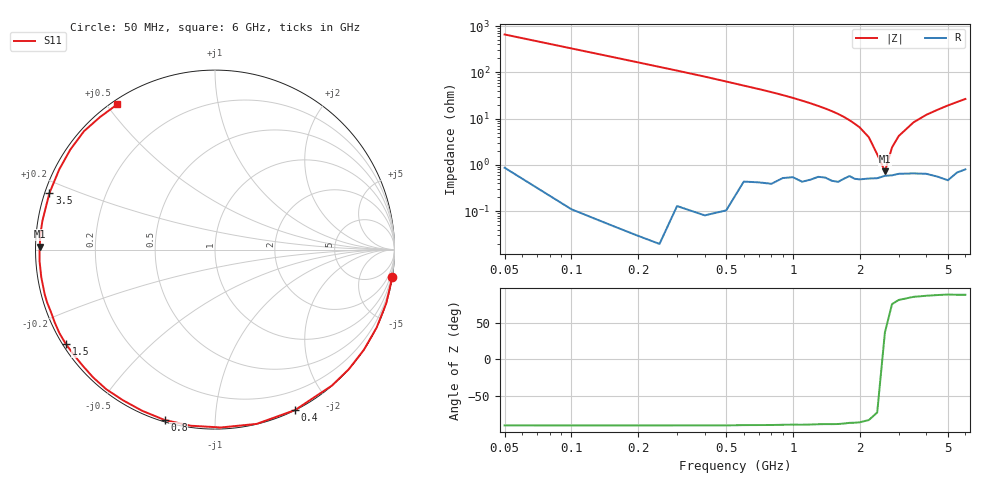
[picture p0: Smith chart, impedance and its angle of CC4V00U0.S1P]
! Infineon Technologies  Discrete & RF Semiconductors
! BBY57-02W
! Si Tuning Diode in SCD-80
! VR = 4 V
! S-Parameters:  June  2000
# GHz  S  MA  R  50
!  f  S11
! GHz  MAG  ANG
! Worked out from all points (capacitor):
!   34 points, 50 MHz to 6 GHz, reference 50 ohm
!   read as one part to ground: C = 4.83 pF near 50 MHz
!   lowest |Z| = 727 mohm at 2.6 GHz (marker M1)
!   series resonance near 2.557 GHz, so ESL is about 800 pH
!   S11 on the Smith chart (normalised r, x): 50 MHz: 0, -13; 400 MHz: 0.00, -1.62; 800 MHz: 0.01, -0.75; 1.5 GHz: 0.01, -0.29; 3.5 GHz: 0.01, +0.17; 6 GHz: 0.02, +0.53
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0.05  0.9998 -8.7
0.1  0.9999 -17.3
0.15  0.9999 -25.7
0.2  0.9999 -33.9
0.25  0.9999 -41.8
0.3  0.9991 -49.3
0.4  0.9991 -63.5
0.5  0.9984 -76.6
0.6  0.9916 -88.1
0.7  0.9905 -97.8
0.8  0.99 -106.5
0.9  0.9854 -114.4
1  0.9836 -121.5
1.1  0.9861 -127.9
1.3  0.9808 -138.8
1.5  0.9834 -147.7
1.6  0.9839 -151.7
1.8  0.978 -159.1
2  0.981 -165.3
2.4  0.9796 -176.3
2.6  0.977 179.0
3  0.9748 170.5
3.5  0.9748 161.2
4  0.976 152.8
4.5  0.9799 145.4
5  0.9839 137.9
5.5  0.9776 130.9
6  0.9753 124.0
